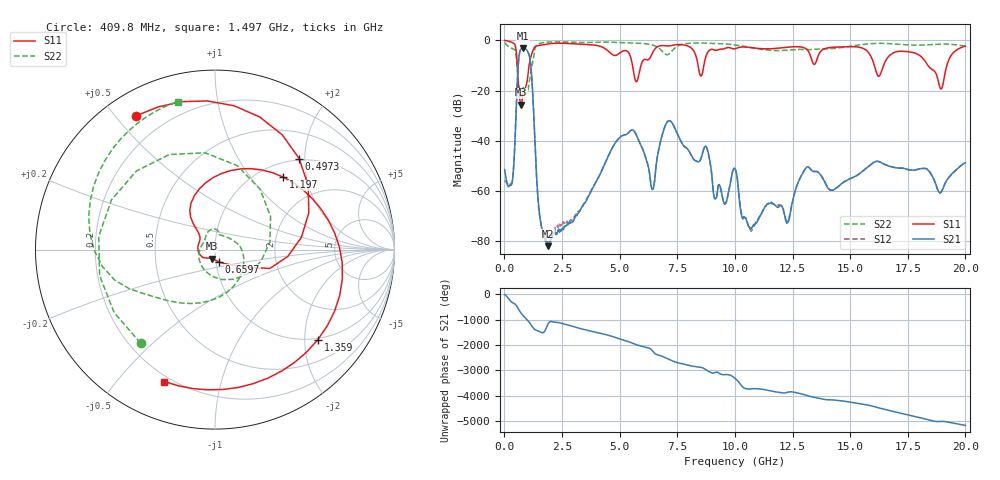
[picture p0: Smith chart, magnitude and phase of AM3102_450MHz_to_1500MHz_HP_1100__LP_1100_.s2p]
!Agilent Technologies,E8364B,MY43040894,A.07.50.67
!Agilent E8364B: A.07.50.67
!Date: Thursday, January 11, 2018 06:35:37
!Correction: S11(Full 2 Port(1,2))
!S21(Full 2 Port(1,2))
!S12(Full 2 Port(1,2))
!S22(Full 2 Port(1,2))
!S2P File: Measurements: S11, S21, S12, S22:
# Hz S  dB  R 50
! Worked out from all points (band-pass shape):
!   1601 points, 10 MHz to 20 GHz, reference 50 ohm
!   highest |S21| = -3.13 dB at 809.6 MHz (marker M1); lowest = -81.9 dB at 1.897 GHz (marker M2)
!   |S21| within 3 dB of the highest: 640 MHz to 1.081 GHz (441.5 MHz wide, 51.3 % of centre)
!   lowest |S11| = -25.6 dB at 722.1 MHz (marker M3), VSWR 1.11, Z = 48.2 - j4.83 ohm
!   |S11| at or under -10 dB: 560.5 MHz to 1.07 GHz (509.2 MHz wide, 62.5 % of centre); 16.05 GHz to 16.45 GHz (400.9 MHz wide, 2.47 % of centre); 18.38 GHz to 19.2 GHz (820.1 MHz wide, 4.37 % of centre)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
!   |S22| runs from -22.4 to -0.6 dB; largest |S21 - S12| = 0.002
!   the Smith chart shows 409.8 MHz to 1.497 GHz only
!   S11 on the Smith chart (normalised r, x): 409.8 MHz: 0.10, +0.57; 497.3 MHz: 0.97, +1.88; 659.7 MHz: 1.04, -0.14; 1.197 GHz: 1.27, +1.48; 1.359 GHz: 0.97, -2.31; 1.497 GHz: 0.17, -0.67
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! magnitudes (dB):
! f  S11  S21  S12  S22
! 10 MHz  -0.1  -51.4  -55.8  -1.0
! 409.8 MHz  -1.3  -49.3  -49.2  -3.5
! 497.3 MHz  -3.2  -30.8  -30.9  -5.3
! 659.7 MHz  -22.9  -4.9  -4.9  -20.7
! 722.1 MHz  -25.6  -3.4  -3.4  -22.2
! 809.6 MHz  -20.5  -3.1  -3.1  -18.9
! 1.197 GHz  -5.1  -16.0  -16.0  -10.2
! 1.359 GHz  -2.4  -47.4  -47.4  -2.5
! 1.497 GHz  -2.1  -66.6  -67.8  -1.4
! 1.897 GHz  -1.4  -81.9  -79.9  -0.7
! 3.346 GHz  -1.6  -66.5  -66.6  -0.9
! 5.045 GHz  -4.8  -38.3  -38.3  -0.9
! 6.419 GHz  -5.2  -59.3  -59.2  -1.9
! 6.682 GHz  -2.4  -44.0  -44.0  -3.0
! 8.743 GHz  -6.4  -42.2  -42.2  -1.2
! 9.568 GHz  -3.3  -65.1  -65.1  -1.5
! 10.01 GHz  -3.4  -51.0  -51.0  -1.9
! 10.7 GHz  -2.9  -74.8  -75.9  -2.9
! 13.34 GHz  -8.0  -51.9  -51.9  -3.6
! 16.68 GHz  -6.4  -50.0  -49.9  -1.3
! 18.94 GHz  -19.4  -60.6  -60.3  -1.5
! 20 GHz  -2.3  -48.7  -48.7  -2.3
